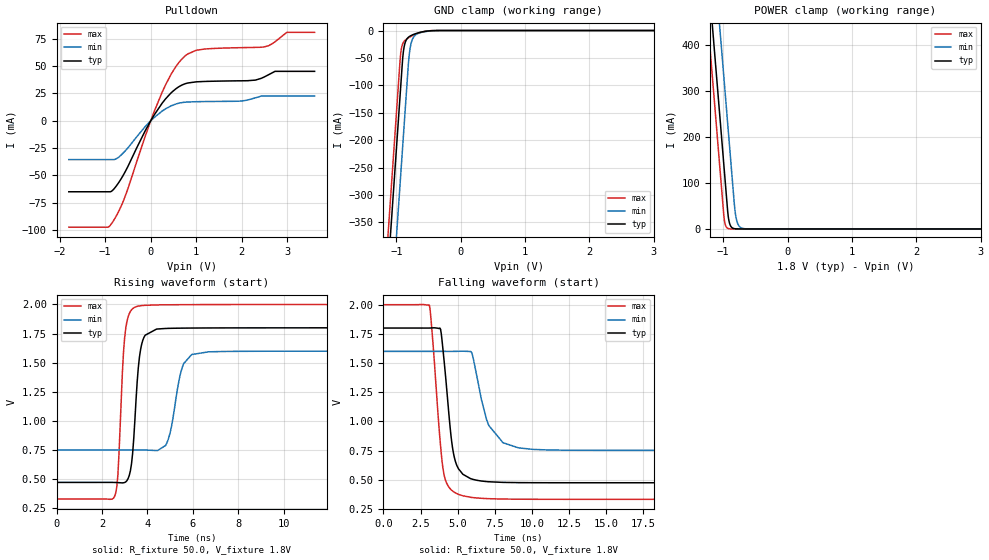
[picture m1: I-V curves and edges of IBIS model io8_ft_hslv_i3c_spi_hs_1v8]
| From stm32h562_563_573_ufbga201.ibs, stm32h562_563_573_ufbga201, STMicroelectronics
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[Model]   io8_ft_hslv_i3c_spi_hs_1v8
Model_type I/O_open_drain
Polarity   Non-Inverting
Enable   Active-Low
| CAP_THRESHOLD on pad IOFT is "UDTCAPC" :
| Rising=20.0% of vddiom   Falling=80.0% of vddiom
| C_comp min and max val. don't necessarily correlate with the min and max pvt
| but are the smallest and greatest pad capacitance found.
| var   typ   min   max
C_comp   3.75311pF  3.69067pF  3.87717pF
|C_comp_pulldown   3.75311pF  3.69067pF  3.87717pF
Vinl = 800.0mV
Vinh = 1.0V
Vmeas = 900.0mV   | Reference voltage for timing measurements
Cref  = 50.0pF   | Timing specification test load capacitance value
Rref  = 1.0MOhm   | Timing specification test load resistance value
Vref  = 990.0mV   | Timing specification test load voltage
[Model Spec]
| TIME_THRESHOLD on pin ZII2CV11 is "CMOS" :
| Rising=40.0% of vdd   Falling=60.0% of vdd
Vinl 703.80000mV 631.80000mV 784.80000mV
Vinh 1.06220V 937.20000mV 1.16620V
| variable   typ   min   max
[Temperature Range] 25.0 125.0 -40.0
| variable   typ   min   max
[Voltage Range] 1.8V 1.6V 2.0V
| variable   typ   min   max
[POWER Clamp Reference] 1.8V 1.6V 2.0V
| variable   typ   min   max
[GND Clamp Reference] 0V 0V 0V
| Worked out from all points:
|   slope of the pulldown table from 0 to 0.27 V, typ, clamps not added: 15.8 ohm
|   GND clamp passes 1 mA (typ) near -0.52 V on its own axis
|   POWER clamp passes 1 mA (typ) near -0.84 V on its own axis
|   rising waveform, R_fixture 50.0, V_fixture 1.8V: 20-80 % time 286ps typ, 464ps min, 244ps max; typ from 0.474 V to 1.8 V
|   falling waveform, R_fixture 50.0, V_fixture 1.8V: 20-80 % time 626ps typ, 1.15ns min, 606ps max; typ from 1.8 V to 0.474 V
[POWER Clamp]
-1.8V     1.518A     1.709A     1.407A
-1.23V    548.8mA    740.2mA    437.5mA
-1.16V    429.8mA    621.2mA    318.5mA
-1.05V    242.8mA    434.2mA    131.5mA
-980mV    123.8mA    315.2mA    17.95mA
-930mV    38.81mA    230.2mA    1.49mA
-910mV    17.82mA    196.2mA    550.8uA
-890mV    8.18mA     162.2mA    203.5uA
-810mV    363.5uA    33.6mA     3.797uA
-770mV    76.62uA    10.47mA    518.8nA
-710mV    7.416uA    1.822mA    26.34nA
3.6V      0A         0A         0A
[GND Clamp]
-1.8V     -1.579A    -1.74A     -1.515A
-1.24V    -627.3mA   -788.3mA   -562.7mA
-1.05V    -304.3mA   -465.3mA   -239.7mA
-940mV    -117.3mA   -278.3mA   -52.69mA
-930mV    -100.3mA   -261.3mA   -40.52mA
-900mV    -50.11mA   -210.3mA   -24.23mA
-880mV    -30.95mA   -176.3mA   -20.02mA
-810mV    -12.18mA   -57.97mA   -13.23mA
-780mV    -9.807mA   -29.1mA    -11.19mA
-690mV    -5.41mA    -7.142mA   -6.184mA
-420mV    -170.4uA   -446.1uA   -81.94uA
3.6V      5.755nA    953.4nA    228.2pA
| variable   typ   min   max
[Pullup Reference] 1.8V 1.6V 2.0V
| variable   typ   min   max
[Pulldown Reference] 0V 0V 0V
[Pulldown]
-1.8V     -65.02mA   -35.56mA   -97.42mA
-940mV    -65.02mA   -35.56mA   -97.42mA
-850mV    -64.17mA   -35.56mA   -93.49mA
-570mV    -47.32mA   -28.01mA   -70.04mA
-120mV    -9.088mA   -5.279mA   -14.07mA
250mV     16.04mA    8.832mA    26.05mA
550mV     29.17mA    15.25mA    49.41mA
780mV     34.17mA    17.07mA    60.14mA
1.18V     35.97mA    17.56mA    65.65mA
2.49V     40mA       22.62mA    67.56mA
2.99V     45.21mA    22.62mA    80.94mA
3.6V      45.21mA    22.62mA    80.94mA
[Ramp]
dV/dt_r 795.76528mV/284.26864ps 508.9493mV/462.32385ps 1.00097V/239.67875ps
dV/dt_f 795.7872mV/625.44325ps 508.98193mV/1.04297ns 1.00099V/604.97502ps
R_load = 50.0
| Removed startup time: 0s 0s 0s  .
| Removed end time: 36.4ns.
[Rising Waveform]
R_fixture   = 50.0
V_fixture   = 1.8V
V_fixture_min = 1.6V
V_fixture_max = 2.0V
0s        473.7mV    751.7mV    331.7mV
2.55ns    473.4mV    751.8mV    351.2mV
2.7ns     472.2mV    751.9mV    535.8mV
3.05ns    478.6mV    752.1mV    1.8V
3.3ns     632mV      752.1mV    1.954V
3.6ns     1.459V     752.1mV    1.986V
4.8ns     1.794V     790.5mV    1.997V
5.6ns     1.797V     1.494V     1.998V
6.7ns     1.799V     1.594V     1.999V
36.4ns    1.8V       1.6V       2V
| Removed startup time: 0s 0s 0s  .
| Removed end time: 49.4ns.
[Falling Waveform]
R_fixture   = 50.0
V_fixture   = 1.8V
V_fixture_min = 1.6V
V_fixture_max = 2.0V
0s        1.8V       1.6V       2V
3.1ns     1.8V       1.6V       1.994V
3.85ns    1.789V     1.6V       787.9mV
4.05ns    1.565V     1.6V       564.8mV
4.65ns    777.4mV    1.6V       403.9mV
5.35ns    546.5mV    1.602V     362.1mV
5.95ns    505.9mV    1.587V     347.9mV
7.1ns     482.3mV    964mV      337.2mV
9.1ns     474.9mV    772.7mV    332.7mV
49.4ns    473.7mV    751.7mV    331.7mV
